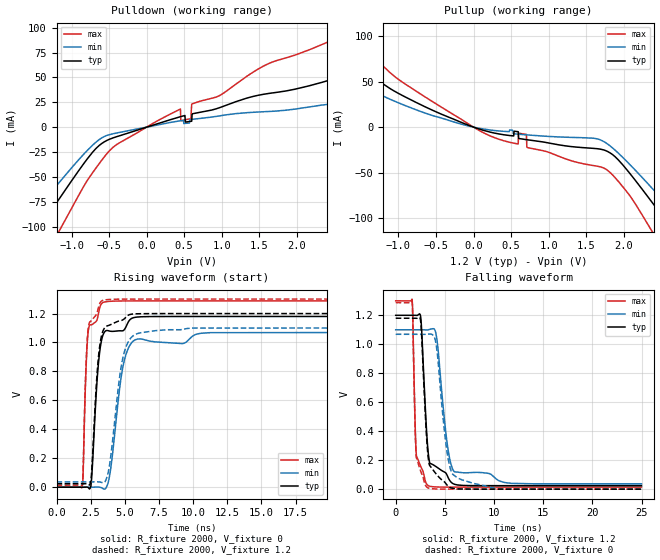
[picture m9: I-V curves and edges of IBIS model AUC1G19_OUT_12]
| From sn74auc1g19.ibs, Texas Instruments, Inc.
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[Model]   AUC1G19_OUT_12
Model_type  Output
Vref =   0
Rref =   2000
Cref =   15p
Vmeas =   0.6
| variable   typ   min   max
C_comp   5.68pF   2.57pF   16.19pF
| C_pullup   5.68pF   2.57pF   16.19pF
| C_pulldown   5.68pF   2.57pF   16.19pF
[Temperature Range]   40   100   -40
| Ambient temperature   25   85   -40
[Voltage range]   1.2   1.1   1.3
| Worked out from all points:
|   slope of the pulldown table from 0 to 0.18 V, typ, clamps not added: 42.2 ohm
|   slope of the pullup table from 0 to 0.18 V, typ, clamps not added: 38.7 ohm
|   rising waveform, R_fixture 2000, V_fixture 0: 20-80 % time 496ps typ, 831ps min, 282ps max; typ from 0 V to 1.18 V
|   falling waveform, R_fixture 2000, V_fixture 1.2: 20-80 % time 565ps typ, 968ps min, 285ps max; typ from 1.2 V to 0.024 V
|   rising waveform, R_fixture 2000, V_fixture 1.2: 20-80 % time 486ps typ, 825ps min, 276ps max; typ from 0.024 V to 1.2 V
|   falling waveform, R_fixture 2000, V_fixture 0: 20-80 % time 562ps typ, 976ps min, 283ps max; typ from 1.18 V to 0 V
[Pulldown]
| AUC1G19_OUT_12
|   Voltage   I(typ)   I(min)   I(max)
-3.6V     -342.1mA   -285.3mA   -424.3mA
-1.81V    -143.9mA   -115.1mA   -191mA
-1.485V   -107.7mA   -84.82mA   -147.8mA
-1.225V   -78.78mA   -61.03mA   -112.7mA
-675mV    -21.46mA   -15.09mA   -41.13mA
-395mV    -9.496mA   -5.836mA   -17.3mA
450mV     10.5mA     6.398mA    18.24mA
590mV     5.848mA    7.731mA    8.546mA
605mV     12.96mA    7.861mA    23.36mA
2.86V     55.96mA    19.1mA     100.7mA
3.42V     44.59mA    20.07mA    119mA
7.2V      57.06mA    26.83mA    107.6mA
[Pullup]
| AUC1G19_OUT_12
|   Voltage   I(typ)   I(min)   I(max)
-3.6V     224mA      100.3mA    290.4mA
-2.705V   158.6mA    66.22mA    205mA
-2.115V   110.4mA    78.06mA    148.8mA
-1.68V    77.78mA    55.72mA    108.5mA
-1.025V   38.18mA    27.56mA    53.97mA
50mV      -1.427mA   -842.9uA   -2.489mA
700mV     -13.68mA   -8.451mA   -7.891mA
1.78V     -26.5mA    -18.21mA   -47.11mA
2.4V      -84.95mA   -69.01mA   -117.5mA
2.695V    -117.7mA   -96.03mA   -157.9mA
3.045V    -157mA     -128.8mA   -205.5mA
7.2V      -622.7mA   -529mA     -757.6mA
[Ramp]
| AUC1G19_OUT_12
| variable   typ   min   max
dV/dt_r   0.72/4.98E-10   0.65/8.41E-10   0.78/2.83E-10
dV/dt_f   0.71/5.72E-10   0.64/9.74E-10   0.78/2.87E-10
R_load = 2000
[Rising Waveform]
| AUC1G19_OUT_12
R_fixture =   2000
C_fixture =   0
L_fixture =   0
V_fixture =   0
V_fixture_min = 0
V_fixture_max = 0
|   Time   V(typ)   V(min)   V(max)
0s        6.566nV    27.84nV    704.7pV
1.89ns    -18.11uV   436.4nV    8.98mV
2.22ns    861.1uV    -8.433uV   947.4mV
2.5ns     2.361mV    -63.84uV   1.122V
3.02ns    802.6mV    896uV      1.177V
3.4ns     1.052V     -9.137mV   1.276V
3.9ns     1.079V     87.05mV    1.284V
4.905ns   1.083V     852.9mV    1.287V
5.735ns   1.174V     1.018V     1.287V
24.99ns   1.18V      1.069V     1.287V
[Falling Waveform]
| AUC1G19_OUT_12
R_fixture =   2000
C_fixture =   0
L_fixture =   0
V_fixture =   1.2
V_fixture_min = 1.1
V_fixture_max = 1.3
|   Time   V(typ)   V(min)   V(max)
0s        1.2V       1.1V       1.3V
1.66ns    1.2V       1.1V       1.312V
1.73ns    1.2V       1.1V       1.219V
2.07ns    1.2V       1.1V       268.5mV
2.51ns    1.202V     1.1V       162.7mV
3.275ns   275mV      1.1V       26.04mV
4.12ns    154.7mV    1.065V     15.42mV
5.235ns   95.56mV    316.1mV    14.13mV
5.955ns   34.44mV    121.2mV    14mV
24.99ns   24.01mV    36.66mV    13.87mV
[Rising Waveform]
| AUC1G19_OUT_12
R_fixture =   2000
C_fixture =   0
L_fixture =   0
V_fixture =   1.2
V_fixture_min = 1.1
V_fixture_max = 1.3
|   Time   V(typ)   V(min)   V(max)
0s        23.98mV    36.64mV    13.86mV
1.88ns    23.96mV    36.64mV    20.87mV
2.21ns    24.85mV    36.63mV    955.6mV
2.47ns    27.42mV    36.6mV     1.145V
2.995ns   818.3mV    37.19mV    1.215V
3.325ns   1.058V     32.69mV    1.288V
3.86ns    1.119V     140.7mV    1.297V
4.86ns    1.157V     895.4mV    1.3V
5.74ns    1.198V     1.054V     1.3V
24.99ns   1.2V       1.1V       1.3V
[Falling Waveform]
| AUC1G19_OUT_12
R_fixture =   2000
C_fixture =   0
L_fixture =   0
V_fixture =   0
V_fixture_min = 0
V_fixture_max = 0
|   Time   V(typ)   V(min)   V(max)
0s        1.18V      1.069V     1.287V
1.66ns    1.18V      1.069V     1.298V
2.06ns    1.179V     1.069V     260.3mV
2.505ns   1.174V     1.069V     131mV
3.195ns   304.4mV    1.069V     12.59mV
3.42ns    169mV      1.071V     6.045mV
4.05ns    110.5mV    1.022V     1.56mV
5.235ns   27.27mV    250.6mV    244.6uV
6.135ns   3.098mV    85.18mV    115.7uV
24.99ns   29.2uV     6.127uV    11.17uV
